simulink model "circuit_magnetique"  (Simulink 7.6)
settings: Solver=ode23tb  StartTime=0.0  StopTime=0.2  RelTol=1e-3
InitFcn:
  | N=1200;
StopFcn:
  | close all
  | load V_Nphi.mat
  | plot(x(1,:),x(2,:),x(1,:),x(3,:))
  | grid
  | axis([0 0.2 -0.04 0.04])
  | title('Tension et N \phi/dt')
  | xlabel('temps')
  | 
  | figure
  | 
  | load NI_MMF.mat
  | plot(y(1,:),y(2,:),y(1,:),y(3,:))
  | grid
  | axis([0 0.2 -300 300])
  | title('Tension et N \phi/dt')
  | xlabel('temps')
libraries: fl_lib x12, nesl_utility x6

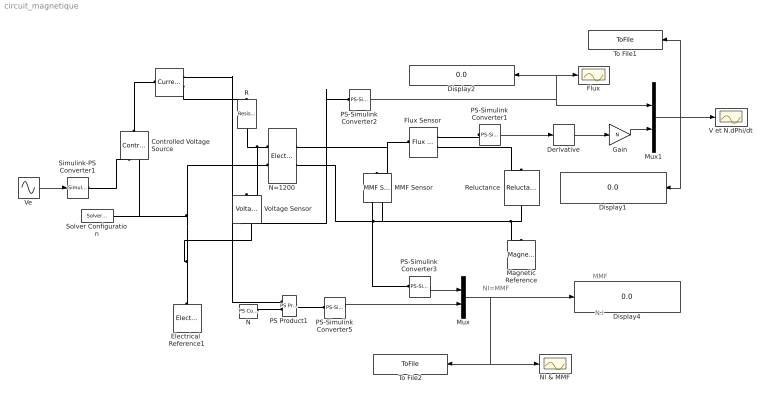
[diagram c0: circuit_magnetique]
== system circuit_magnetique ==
  note: NI=MMF
  note: MMF
  note: N.I
  Controlled Voltage Source : fl_lib/Electrical/Electrical Sources/Controlled Voltage Source  DialogController=NetworkEngine.DynNeDlgSource  SystemSampleTime=-1  i_Log=off  v_Log=off  LocalVarNames=|i|v  LocalVarDescs=|i|v  LocalVarLogging=[0 0]
  Derivative : Derivative
  Display1 : Display
  Display2 : Display
  Display4 : Display
  Electrical  Reference1 : fl_lib/Electrical/Electrical Elements/Electrical Reference  DialogController=NetworkEngine.DynNeDlgSource  SystemSampleTime=-1  i_Log=off  LocalVarNames=|i  LocalVarDescs=|i  LocalVarLogging=0
  Flux : Scope
  Flux Sensor : fl_lib/Magnetic/Magnetic Sensors/Flux Sensor  DialogController=NetworkEngine.DynNeDlgSource  SystemSampleTime=-1  phi_Log=off  mmf_Log=off  LocalVarNames=|phi|mmf  LocalVarDescs=|phi|mmf  LocalVarLogging=[0 0]
  Gain : Gain  Gain=N
  I : fl_lib/Electrical/Electrical Sensors/Current Sensor  DialogController=NetworkEngine.DynNeDlgSource  SystemSampleTime=-1  i1_Log=off  v1_Log=off  LocalVarNames=|i1|v1  LocalVarDescs=|i1|v1  LocalVarLogging=[0 0]
  MMF Sensor : fl_lib/Magnetic/Magnetic Sensors/MMF Sensor  DialogController=NetworkEngine.DynNeDlgSource  SystemSampleTime=-1  phi_Log=off  mmf_Log=off  LocalVarNames=|phi|mmf  LocalVarDescs=|phi|mmf  LocalVarLogging=[0 0]
  Magnetic Reference : fl_lib/Magnetic/Magnetic Elements/Magnetic Reference  DialogController=NetworkEngine.DynNeDlgSource  SystemSampleTime=-1  phi_Log=off  LocalVarNames=|phi  LocalVarDescs=|phi  LocalVarLogging=0
  Mux : Mux  Inputs=2
  Mux1 : Mux  Inputs=2
  N : fl_lib/Physical Signals/Sources/PS Constant  DialogController=NetworkEngine.DynNeDlgSource  SystemSampleTime=-1  constant=N  LocalVarLogging=[]
  N=1200 : fl_lib/Magnetic/Magnetic Elements/Electromagnetic Converter  DialogController=NetworkEngine.DynNeDlgSource  SystemSampleTime=-1  Nw=N  i_Log=off  v_Log=off  mmf_Log=off  phi_Log=off  LocalVarNames=|i|v|mmf|phi  LocalVarDescs=|i|v|mmf|phi  LocalVarLogging=[0 0 0 0]
  NI & MMF : Scope
  PS Product1 : fl_lib/Physical Signals/Functions/PS Product  DialogController=NetworkEngine.DynNeDlgSource  SystemSampleTime=-1  LocalVarLogging=[]
  PS-Simulink Converter{1..3,5} (4 alike) : nesl_utility/PS-Simulink Converter  DialogController=NetworkEngine.DynNeUtilDlgSource  SystemSampleTime=-1  PhysicalDomain=network_engine_domain  LeftPortType=input  RightPortType=output  SubClassName=ps_output  Unit=1  AffineConversion=off
  R : fl_lib/Electrical/Electrical Elements/Resistor  DialogController=NetworkEngine.DynNeDlgSource  SystemSampleTime=-1  R=1 kOhm  i_Log=off  v_Log=off  LocalVarNames=|i|v  LocalVarDescs=|i|v  LocalVarLogging=[0 0]
  Reluctance : fl_lib/Magnetic/Magnetic Elements/Reluctance  DialogController=NetworkEngine.DynNeDlgSource  SystemSampleTime=-1  g=0.3 m  CSA=4e-004 m^2  mur=1  phi_Log=off  mmf_Log=off  LocalVarNames=|phi|mmf  LocalVarDescs=|phi|mmf  LocalVarLogging=[0 0]
  Simulink-PS Converter1 : nesl_utility/Simulink-PS Converter  DialogController=NetworkEngine.DynNeUtilDlgSource  SystemSampleTime=-1  PhysicalDomain=network_engine_domain  LeftPortType=input  RightPortType=output  SubClassName=ps_input  Unit=1  AffineConversion=off  InputFilterTimeConstant=.001  UdotUserProvided=0
  Solver Configuration : nesl_utility/Solver Configuration  DialogController=NetworkEngine.DynNeUtilDlgSource  SystemSampleTime=-1  PhysicalDomain=network_engine_domain  LeftPortType=input  RightPortType=generic  SubClassName=solver  Accelerate=off  Profile=off  ResidualTolerance=1e-9  MaxNonlinIter=3  MaxModeIter=2  DoFixedCost=off  UseLocalSampling=off  DoDC=off  LinearAlgebra=Sparse  LocalSolverSampleTime=.001  LocalSolverChoice=NE_BACKWARD_EULER_ADVANCER  UseLocalSolver=off
  To File1 : ToFile  Filename=V_Nphi  MatrixName=x
  To File2 : ToFile  Filename=NI_MMF  MatrixName=y
  V et N.dPhi/dt : Scope
  Ve : Sin  Amplitude=220  Frequency=60  Phase=pi/2  SampleTime=0
  Voltage Sensor : fl_lib/Electrical/Electrical Sensors/Voltage Sensor  DialogController=NetworkEngine.DynNeDlgSource  SystemSampleTime=-1  i1_Log=off  v1_Log=off  LocalVarNames=|i1|v1  LocalVarDescs=|i1|v1  LocalVarLogging=[0 0]
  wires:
  Ve/1 -> Simulink-PS Converter1/1
  PS-Simulink Converter3/1 -> Mux/1
  PS-Simulink Converter1/1 -> Derivative/1
  PS-Simulink Converter5/1 -> Mux/2
  Mux/1 -> Display4/1, NI & MMF/1, To File2/1
  Derivative/1 -> Gain/1
  Mux1/1 -> V et N.dPhi/dt/1, Display1/1, To File1/1
  PS-Simulink Converter2/1 -> Mux1/1, Flux/1, Display2/1
  Gain/1 -> Mux1/2
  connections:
  Flux Sensor/LConn1 -- N=1200/RConn1 -- MMF Sensor/LConn1
  Simulink-PS Converter1/RConn1 -- Controlled Voltage Source/RConn1
  Controlled Voltage Source/LConn1 -- I/LConn1
  Electrical  Reference1/LConn1 -- Controlled Voltage Source/RConn2 -- Solver Configuration/RConn1 -- N=1200/LConn2 -- Voltage Sensor/RConn2
  MMF Sensor/RConn1 -- PS-Simulink Converter3/LConn1
  PS-Simulink Converter1/LConn1 -- Flux Sensor/RConn1
  I/RConn2 -- R/LConn1
  N=1200/LConn1 -- R/RConn1 -- Voltage Sensor/LConn1
  N/RConn1 -- PS Product1/LConn2
  PS Product1/RConn1 -- PS-Simulink Converter5/LConn1
  PS Product1/LConn1 -- I/RConn1
  Flux Sensor/RConn2 -- Reluctance/LConn1
  N=1200/RConn2 -- Reluctance/RConn1 -- Magnetic Reference/LConn1 -- MMF Sensor/RConn2
  Voltage Sensor/RConn1 -- PS-Simulink Converter2/LConn1
